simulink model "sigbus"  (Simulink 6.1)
settings: Solver=ode45  StartTime=0.0  StopTime=10.0  RelTol=1e-3

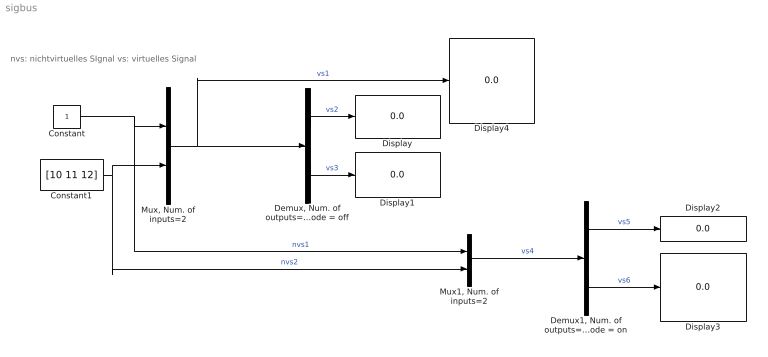
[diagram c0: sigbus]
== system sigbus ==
  note: nvs: nichtvirtuelles SIgnal vs: virtuelles Signal
  Constant : Constant
  Constant1 : Constant  Value=[10 11 12]
  "Demux, Num. of outputs=2, Bus selection mode = off" : Demux  Outputs=2
  "Demux1, Num. of outputs=2, Bus selection mode = on" : Demux  Outputs=2  BusSelectionMode=on
  Display{,1..4} (5 alike) : Display
  "Mux, Num. of inputs=2" : Mux  Inputs=2
  "Mux1, Num. of inputs=2" : Mux  Inputs=2
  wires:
  Constant/1 -> "Mux, Num. of inputs=2"/1, "Mux1, Num. of inputs=2"/1  "nvs1"
  Constant1/1 -> "Mux, Num. of inputs=2"/2, "Mux1, Num. of inputs=2"/2  "nvs2"
  "Mux, Num. of inputs=2"/1 -> "Demux, Num. of outputs=2, Bus selection mode = off"/1, Display4/1  "vs1"
  "Demux, Num. of outputs=2, Bus selection mode = off"/1 -> Display/1  "vs2"
  "Demux, Num. of outputs=2, Bus selection mode = off"/2 -> Display1/1  "vs3"
  "Demux1, Num. of outputs=2, Bus selection mode = on"/1 -> Display2/1  "vs5"
  "Demux1, Num. of outputs=2, Bus selection mode = on"/2 -> Display3/1  "vs6"
  "Mux1, Num. of inputs=2"/1 -> "Demux1, Num. of outputs=2, Bus selection mode = on"/1  "vs4"
